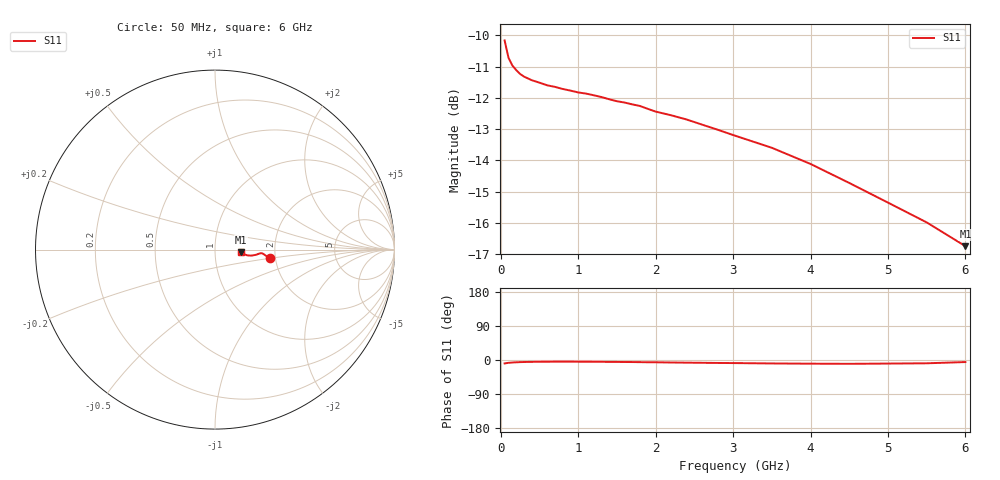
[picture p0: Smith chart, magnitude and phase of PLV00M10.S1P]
! Infineon Technologies  Discrete & RF Semiconductors
! BAR 64-04W /-05W /-06W
! Si PIN Diode in SOT323
! IF = 0.1 mA
! S-Parameters:  October  2008
# GHz  S  MA  R  50
!  f  S11
! GHz  MAG  ANG
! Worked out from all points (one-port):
!   34 points, 50 MHz to 6 GHz, reference 50 ohm
!   lowest |S11| = -16.7 dB at 6 GHz (marker M1), VSWR 1.34, Z = 66.9 - j1.87 ohm
!   |S11| at or under -10 dB: start of sweep to end of sweep
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0.05  0.3103 -9.1
0.1  0.2912 -7.4
0.15  0.283 -6.6
0.2  0.2783 -6.0
0.25  0.2743 -5.6
0.3  0.2717 -5.3
0.4  0.2681 -4.9
0.6  0.2631 -4.6
0.7  0.2616 -4.4
0.8  0.2596 -4.4
1  0.2563 -4.5
1.1  0.2552 -4.6
1.2  0.2537 -4.7
1.3  0.252 -4.8
1.5  0.2482 -5.1
1.6  0.2469 -5.3
1.7  0.2453 -5.4
1.8  0.2438 -5.7
2  0.2389 -6.0
2.2  0.2356 -6.6
2.4  0.232 -7.0
3  0.2191 -8.1
3.5  0.2091 -9.1
4  0.197 -9.7
4.5  0.1837 -10.1
5  0.1709 -9.4
5.5  0.1589 -8.7
6  0.1456 -5.4
